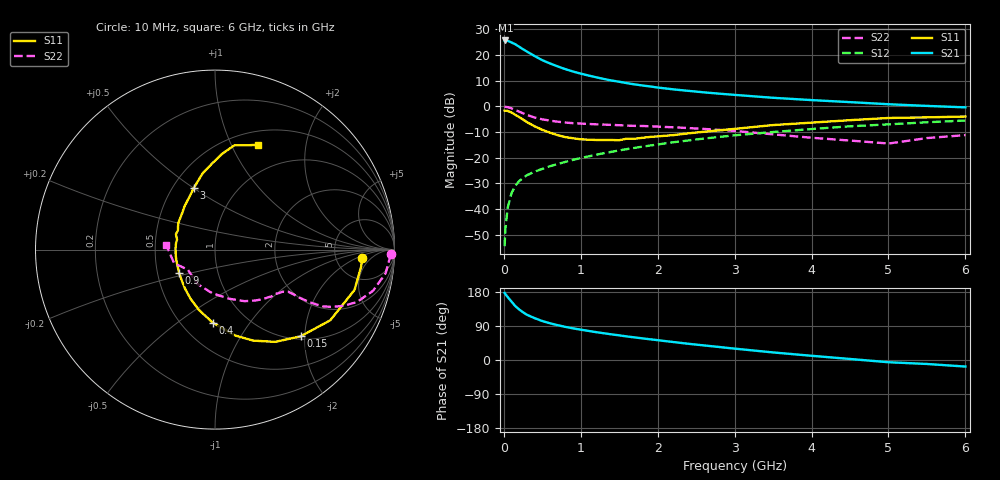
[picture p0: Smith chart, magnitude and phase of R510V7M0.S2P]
! SIEMENS Small Signal Semiconductors
! BFR183
! Si NPN RF Bipolar Junction Transistor in SOT23
! VCE = 10 V  IC = 7 mA
! Common Emitter S-Parameters:  May  1996
# GHz  S  MA  R  50
!  f  S11  S21  S12  S22
! GHz  MAG  ANG  MAG  ANG  MAG  ANG  MAG  ANG
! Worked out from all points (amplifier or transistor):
!   36 points, 10 MHz to 6 GHz, reference 50 ohm
!   highest |S21| = 25.6 dB at 20 MHz (marker M1)
!   |S21| within 3 dB of that: start of sweep to 227.7 MHz
!   unconditionally stable (mu >= 1): 968.2 MHz to 2.735 GHz
!   at 250 MHz: K = 0.50, MSG = 25.0 dB, |S12| = -27.8 dB
!   at 1.4 GHz: K = 1.05, MAG = 12.5 dB, |S12| = -17.7 dB
!   at 6 GHz: K = 0.88, MSG = 2.6 dB, |S12| = -5.6 dB
!   S11 on the Smith chart (normalised r, x): 10 MHz: 9.45, -2.77; 150 MHz: 1.06, -1.90; 400 MHz: 0.70, -0.68; 900 MHz: 0.65, -0.18; 3 GHz: 0.63, +0.50; 6 GHz: 0.65, +1.27
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0.01  0.8226 -3.3  18.81 176.9  0.0019 84.9  0.9805 -1.5
0.02  0.8196 -6.7  19 173.9  0.0041 86.9  0.9736 -3.1
0.05  0.8092 -16.1  18.66 166.1  0.0106 79.9  0.9598 -7.9
0.1  0.7535 -31.5  17.38 154.0  0.0205 74.3  0.9099 -14.6
0.15  0.6789 -45.4  15.98 142.0  0.0286 68.2  0.8441 -20.2
0.2  0.6136 -56.9  14.31 133.4  0.035 65.4  0.7823 -23.6
0.25  0.5501 -67.2  12.79 125.8  0.0407 61.9  0.7262 -26.1
0.3  0.4918 -76.8  11.56 119.4  0.0455 60.8  0.6774 -27.8
0.4  0.4067 -91.9  9.455 110.4  0.0534 59.5  0.6029 -29.1
0.5  0.3478 -104.9  7.851 102.8  0.0604 59.7  0.5557 -29.5
0.6  0.3057 -116.5  6.782 96.9  0.0682 59.8  0.5242 -29.7
0.7  0.2732 -127.9  5.949 91.8  0.0751 60.7  0.5002 -29.7
0.9  0.2382 -147.4  4.724 83.5  0.0906 61.4  0.4683 -29.9
1.1  0.2235 -165.3  3.953 76.8  0.1058 61.6  0.452 -31.3
1.3  0.2201 178.5  3.388 70.6  0.1221 61.5  0.4387 -32.7
1.6  0.2342 158.5  2.809 62.1  0.1467 60.6  0.4201 -35.8
2.2  0.274 131.8  2.13 47.5  0.1988 57.2  0.3895 -44.3
3  0.3628 109.0  1.662 30.0  0.2717 49.9  0.3307 -60.3
3.5  0.4298 99.3  1.459 20.0  0.315 44.2  0.284 -74.3
4.5  0.5354 85.7  1.201 2.7  0.4072 32.8  0.2149 -117.2
5.5  0.6072 73.1  1.014 -10.5  0.4875 21.3  0.2402 -161.5
6  0.6304 67.9  0.95 -17.3  0.527 13.7  0.2743 174.1
